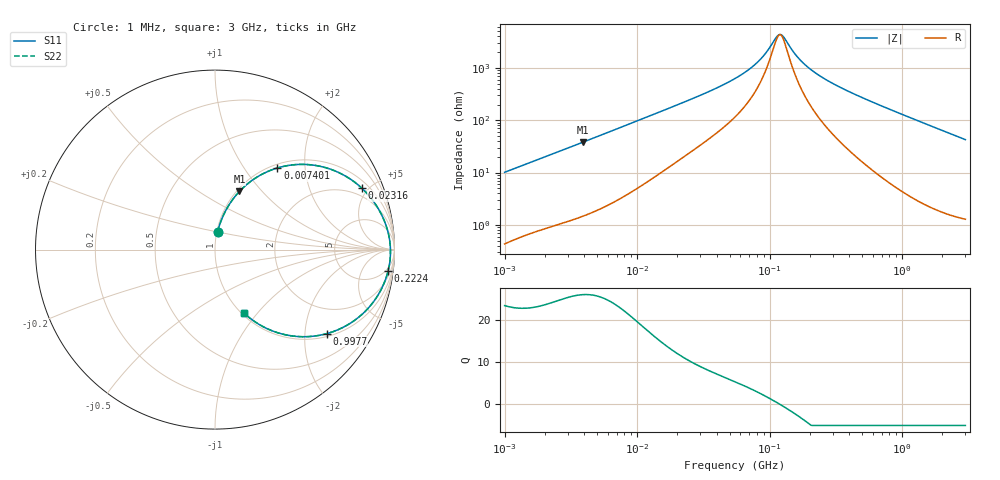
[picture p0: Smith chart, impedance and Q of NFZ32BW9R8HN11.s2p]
! NFZ32BW9R8HN11
# Hz S RI R 50
!Freq.(Hz) S11(Real) S11(Imag) S21(Real) S21(Imag) S12(Real) S12(Imag) S22(Real) S22(Imag)
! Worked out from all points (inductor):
!   401 points, 1 MHz to 3 GHz, reference 50 ohm
!   read as one part in series: L = 1.6 uH near 1.041 MHz
!   highest Q = 26 at 3.9 MHz (marker M1), where L = 1.55 uH
!   self-resonance near 119.5 MHz
!   S11 on the Smith chart (normalised r, x): 1 MHz: 1.01, +0.20; 7.401 MHz: 1.06, +1.44; 23.16 MHz: 1.42, +4.54; 222.4 MHz: 4, -16; 997.7 MHz: 1.09, -2.59; 3 GHz: 1.03, -0.85
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1000000  0.0143 0.0993  0.9857 -0.0993  0.9857 -0.0993  0.0143 0.0993
2182827  0.0522 0.2024  0.9478 -0.2024  0.9478 -0.2024  0.0522 0.2024
3823119  0.1318 0.3196  0.8682 -0.3196  0.8682 -0.3196  0.1318 0.3196
3900413  0.1362 0.3243  0.8638 -0.3243  0.8638 -0.3243  0.1362 0.3243
7400828  0.3478 0.4549  0.6522 -0.4549  0.6522 -0.4549  0.3478 0.4549
1.040059e7  0.5057 0.4745  0.4943 -0.4745  0.4943 -0.4745  0.5057 0.4745
1.461624e7  0.66 0.4419  0.34 -0.4419  0.34 -0.4419  0.66 0.4419
2.316168e7  0.8172 0.343  0.1828 -0.343  0.1828 -0.343  0.8172 0.343
5.477226e7  0.9495 0.1446  0.0505 -0.1446  0.0505 -0.1446  0.9495 0.1446
8.173662e7  0.9706 0.0679  0.0294 -0.0679  0.0294 -0.0679  0.9706 0.0679
9.402997e7  0.9744 0.0426  0.0256 -0.0426  0.0256 -0.0426  0.9744 0.0426
1.125904e8  0.9772 0.0106  0.0228 -0.0106  0.0228 -0.0106  0.9772 0.0106
1.195584e8  0.9776 -3.71e-05  0.0224 3.71e-05  0.0224 3.71e-05  0.9776 -3.71e-05
1.269575e8  0.9777 -0.0107  0.0223 0.0107  0.0223 0.0107  0.9777 -0.0107
1.680187e8  0.9748 -0.0617  0.0252 0.0617  0.0252 0.0617  0.9748 -0.0617
2.094008e8  0.9678 -0.1045  0.0322 0.1045  0.0322 0.1045  0.9678 -0.1045
2.223601e8  0.965 -0.1167  0.035 0.1167  0.035 0.1167  0.965 -0.1167
3.894533e8  0.9124 -0.2467  0.0876 0.2467  0.0876 0.2467  0.9124 -0.2467
8.005644e8  0.7189 -0.4305  0.2811 0.4305  0.2811 0.4305  0.7189 -0.4305
9.977393e8  0.6233 -0.4681  0.3767 0.4681  0.3767 0.4681  0.6233 -0.4681
1.613037e9  0.3905 -0.4742  0.6095 0.4742  0.6095 0.4742  0.3905 -0.4742
3e9  0.161 -0.3528  0.839 0.3528  0.839 0.3528  0.161 -0.3528
